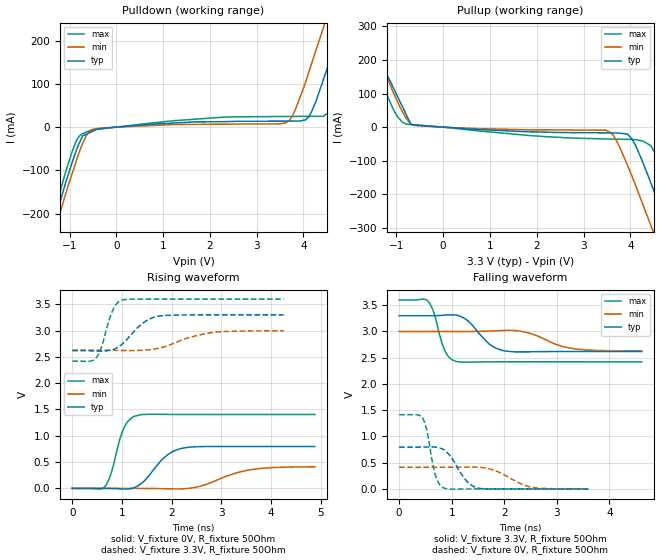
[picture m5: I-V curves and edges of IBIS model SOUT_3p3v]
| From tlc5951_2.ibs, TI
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|   sout_3p3v Model
[Model]   SOUT_3p3v
Model_type   Output
Polarity   Non-Inverting
Enable   Active-Low
Vmeas = 1.65
Vref = 1.65
Cref = 15pF
Rref = 50
|   typ   min   max
|   (nom PVT)   (Fast PVT)   (slow PVT)
|Average
C_comp   1.989e-12   1.632e-12   2.108e-12
|ON state : BUFFER OUTPUT TURNED HIGH
|C_comp   1.989e-12   1.632e-12   2.108e-12
|OFF state: BUFFER OUTPUT TURNED LOW
|C_comp   1.774e-12   1.639e-12   1.805e-12
| Where nom  PVT is Nominal Process,  3.3V,  65C
|   Fast PVT is Strong Process,   3.6V,  -40C
|   Slow PVT is Weak Process,   3V,  125C
[Voltage Range]   3.3   3   3.6
|Ambient Temperature   25   85   -40
|Junction Temperature
[Temperature Range]   65   125   -40
[Pullup Reference]   3.3   3   3.6
[Pulldown Reference]   0   0   0
[Power Clamp Reference]   3.3   3   3.6
[GND Clamp Reference]   0   0   0
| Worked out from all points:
|   slope of the pulldown table from 0 to 0.495 V, typ, clamps not added: 108 ohm
|   slope of the pullup table from 0 to 0.495 V, typ, clamps not added: 107 ohm
|   falling waveform, V_fixture 3.3V, R_fixture 50Ohm: 20-80 % time 373ps typ, 549ps min, 203ps max; typ from 3.3 V to 2.62 V
|   rising waveform, V_fixture 0V, R_fixture 50Ohm: 20-80 % time 450ps typ, 732ps min, 249ps max; typ from 0 V to 0.796 V
|   rising waveform, V_fixture 3.3V, R_fixture 50Ohm: 20-80 % time 435ps typ, 709ps min, 229ps max; typ from 2.62 V to 3.3 V
|   falling waveform, V_fixture 0V, R_fixture 50Ohm: 20-80 % time 313ps typ, 484ps min, 162ps max; typ from 0.796 V to 0 V
[Pulldown]
|   Voltage   I(typ)   I(min)   I(max)
-3.3V     -1.005A    -939.3mA   -1.071A
-1.55V    -306.8mA   -325.2mA   -289.6mA
-1.297V   -207.9mA   -232.6mA   -186.2mA
-848.4mV  -52.02mA   -75.48mA   -30mA
-537mV    -11.12mA   -6.144mA   -7.431mA
3.612V    13.91mA    9.274mA    24.73mA
4.102V    22.6mA     123.2mA    24.89mA
4.426V    110.1mA    230.2mA    25.16mA
4.8V      234mA      352.5mA    109.8mA
5.059V    323.8mA    433.2mA    199.5mA
5.344V    423.1mA    520.5mA    302.1mA
6.6V      852mA      906.2mA    787.9mA
[Pullup]
|   Voltage   I(typ)   I(min)   I(max)
-3.3V     837mA      804.9mA    883.4mA
-1.881V   352.6mA    370.5mA    329.5mA
-1.626V   279mA      288.7mA    237.5mA
-866.4mV  59.6mA     44.8mA     13.86mA
-686.4mV  7.619mA    9.418mA    7.583mA
3.477V    -17.06mA   -9.278mA   -35.14mA
3.937V    -20.58mA   -113.3mA   -36.38mA
4.267V    -105mA     -230.2mA   -41.27mA
4.444V    -168mA     -294.8mA   -56.78mA
4.811V    -309.5mA   -428.1mA   -183.9mA
5.07V     -413.5mA   -520.2mA   -292.1mA
6.6V      -1.024A    -1.055A    -975.8mA
[Ramp]
R_load = 50
|   typ   min   max
dV/dt_r   0.477591/4.4908e-10   0.247444/7.31083e-10   0.843424/2.48832e-10
dV/dt_f   0.409084/3.54504e-10   0.222219/5.42461e-10   0.706864/2.02647e-10
[Falling Waveform]
V_fixture = 3.3V
V_fixture_min = 3V
V_fixture_max = 3.6V
R_fixture = 50Ohm
|   Time   V(typ)   V(min)   V(max)
0s        3.3V       3V         3.6V
546ps     3.3V       3V         3.582V
663ps     3.301V     3V         3.348V
858ps     3.311V     3V         2.662V
1.079ns   3.313V     3V         2.431V
1.703ns   2.77V      3.007V     2.421V
1.976ns   2.637V     3.019V     2.422V
2.418ns   2.611V     2.984V     2.422V
3.367ns   2.618V     2.666V     2.422V
4.615ns   2.618V     2.63V      2.422V
[Rising Waveform]
V_fixture = 0V
V_fixture_min = 0V
V_fixture_max = 0V
R_fixture = 50Ohm
|   Time   V(typ)   V(min)   V(max)
0s        325.2pV    2.121nV    319.2pV
663ps     -606.7uV   277.3uV    43.27mV
780ps     -2.498mV   368.6uV    284.9mV
1.027ns   -10.61mV   355.7uV    1.124V
1.261ns   20.43mV    -264.7uV   1.375V
1.469ns   163.3mV    -1.421mV   1.406V
1.846ns   583.5mV    -6.128mV   1.407V
2.21ns    762.8mV    -8.737mV   1.405V
3.523ns   796mV      344.6mV    1.405V
4.875ns   795.9mV    410.9mV    1.405V
[Rising Waveform]
V_fixture = 3.3V
V_fixture_min = 3V
V_fixture_max = 3.6V
R_fixture = 50Ohm
|   Time   V(typ)   V(min)   V(max)
0s        2.618V     2.63V      2.419V
351ps     2.616V     2.63V      2.417V
481ps     2.611V     2.63V      2.484V
585ps     2.61V      2.629V     2.683V
819ps     2.639V     2.625V     3.396V
1.014ns   2.753V     2.622V     3.584V
1.378ns   3.112V     2.625V     3.599V
1.716ns   3.272V     2.661V     3.6V
2.795ns   3.3V       2.961V     3.6V
4.251ns   3.3V       2.999V     3.6V
[Falling Waveform]
V_fixture = 0V
V_fixture_min = 0V
V_fixture_max = 0V
R_fixture = 50Ohm
|   Time   V(typ)   V(min)   V(max)
0s        796.3mV    412.5mV    1.415V
442ps     797.6mV    412.2mV    1.365V
533ps     799.1mV    412.2mV    1.086V
689ps     796.5mV    412.5mV    267mV
767ps     780.9mV    412.7mV    88.03mV
845ps     748.9mV    413.1mV    20.74mV
1.3ns     131.7mV    417.9mV    -167.7uV
1.508ns   16.95mV    413.7mV    459.7uV
2.535ns   84.74uV    30.05mV    351.1uV
3.601ns   106uV      799.4uV    285uV
